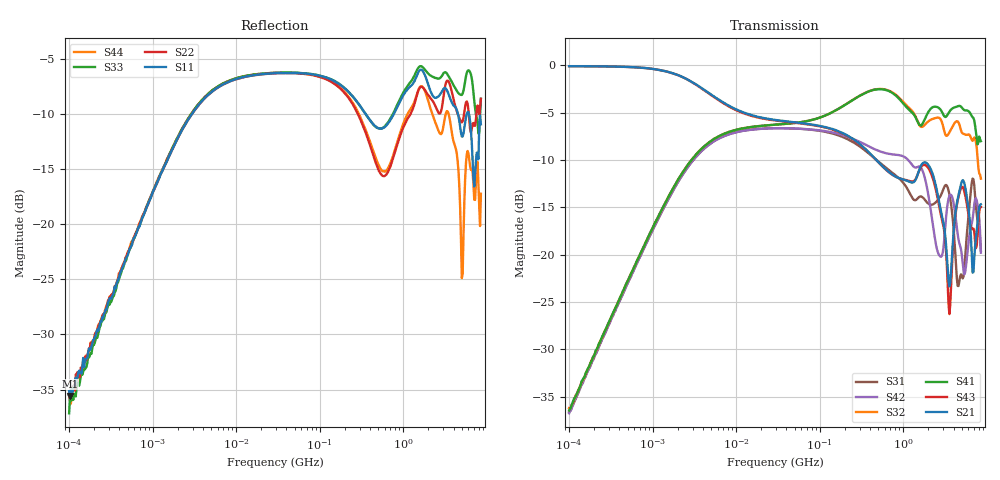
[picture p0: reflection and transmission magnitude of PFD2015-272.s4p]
# MHz S MA R 50
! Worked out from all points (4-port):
!   498 points, 100 kHz to 8.5 GHz, reference 50 ohm
!   strongest paths, dB at 100 kHz, 1.698 MHz, 29.49 MHz, 500.7 MHz, 8.5 GHz:
!     S21: -0.1, -0.8, -5.8, -10.2, -14.7
!     S43: -0.1, -0.8, -5.8, -10.2, -15.0
!     S41: -36.5, -13.2, -6.3, -2.5, -8.0
!     S32: -36.2, -13.2, -6.3, -2.5, -12.0
!     S42: -36.7, -13.5, -6.7, -9.0, -19.8
!     S31: -36.6, -13.5, -6.7, -10.1, -19.6
!   lowest |S11| = -35.6 dB at 102.3 kHz (marker M1), VSWR 1.03, Z = 50.8 + j1.48 ohm
!   |S11| at or under -10 dB: 356.1 MHz to 770.4 MHz (414.3 MHz wide, 73.6 % of centre); 4.523 GHz to 5.754 GHz (1.231 GHz wide, 23.9 % of centre); 6.117 GHz to end of sweep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
0.1  0.01749 61.8  0.9874 -0.8  0.01474 -92.3  0.01505 85.9
     0.9874 -0.8  0.0167 67.2  0.01552 87.9  0.01455 -93.5
     0.01474 -92.3  0.01552 87.9  0.01387 59.1  0.9871 -0.9
     0.01505 85.9  0.01455 -93.5  0.9871 -0.9  0.0167 69.8
0.1023101  0.01662 61.6  0.9874 -0.9  0.01489 -92.3  0.01535 87.0
           0.9874 -0.9  0.01694 69.7  0.01545 87.7  0.01489 -92.2
           0.01489 -92.3  0.01545 87.7  0.01641 60.9  0.9873 -0.9
           0.01535 87.0  0.01489 -92.2  0.9873 -0.9  0.01577 64.9
7.322332  0.4354 23.1  0.6279 -19.7  0.424 -158.1  0.436 24.5
          0.6279 -19.7  0.4348 22.8  0.4365 24.5  0.4238 -158.5
          0.424 -158.1  0.4365 24.5  0.4397 23.0  0.6225 -19.9
          0.436 24.5  0.4238 -158.5  0.6225 -19.9  0.4401 22.6
1248.181  0.4265 -164.8  0.2406 1.7  0.2037 -159.5  0.5673 -172.1
          0.2406 1.7  0.322 -148.7  0.5797 -176.8  0.3012 -165.9
          0.2037 -159.5  0.5797 -176.8  0.4472 -156.7  0.2433 3.0
          0.5673 -172.1  0.3012 -165.9  0.2433 3.0  0.3377 -159.1
2776.003  0.39 -15.9  0.1767 12.2  0.2029 146.7  0.5848 -1.8
          0.1767 12.2  0.32 7.8  0.521 -7.5  0.09767 133.2
          0.2029 146.7  0.521 -7.5  0.4625 0.7  0.1679 20.6
          0.5848 -1.8  0.09767 133.2  0.1679 20.6  0.2573 -14.8
4187.455  0.341 179.4  0.1614 -55.3  0.1036 -141.5  0.5996 179.0
          0.1614 -55.3  0.3443 -175.1  0.4991 179.2  0.1643 -165.9
          0.1036 -141.5  0.4991 179.2  0.4147 178.6  0.1567 -60.5
          0.5996 179.0  0.1643 -165.9  0.1567 -60.5  0.2253 -175.7
8500  0.2842 -46.7  0.1842 44.6  0.1048 23.3  0.397 -34.9
      0.1842 44.6  0.3711 -48.9  0.2518 -21.2  0.1024 -33.6
      0.1048 23.3  0.2518 -21.2  0.3716 -38.4  0.1785 42.6
      0.397 -34.9  0.1024 -33.6  0.1785 42.6  0.1376 -14.9
